VAR_GLOBAL
	
//datapoints SLAVE -> MASTER (monitoring direction)
	(* Input *)

	(* Output *)
	
	(* Memory *)

	(* Data *)
		(*Single Points*)
			// bSlaveToMaster
			bSlaveToMaster 			: BOOL;		// obj addr: 10 - M_SP_NA_1
			nSIQ_bSlaveToMaster 	: BYTE;		// data value and qualifier
			eSPI_bSlaveToMaster		: E_IEC870_5_101SPI;// data value as enum type
			nQDS_bSlaveToMaster		: BYTE;		// data qualifier only
			
	
//datapoints MASTER -> SLAVE (control direction)
	(* Input *)

	(* Output *)
	
	(* Memory *)

	(* Data *)
		(*Single Commands*)
			// bMasterToSlave
			bMasterToSlave 			: BOOL;		// obj addr: 101 - C_SC_NA_1
			nSCO_bMasterToSlave	 	: BYTE;		// command value and qualifier
			eSCS_bMasterToSlave		: E_IEC870_5_101SCS;// command value as enum type
			eQU_bMasterToSlave		: E_IEC870_5_101QU;// command qualifier only
			
	
//other variables	

END_VAR
